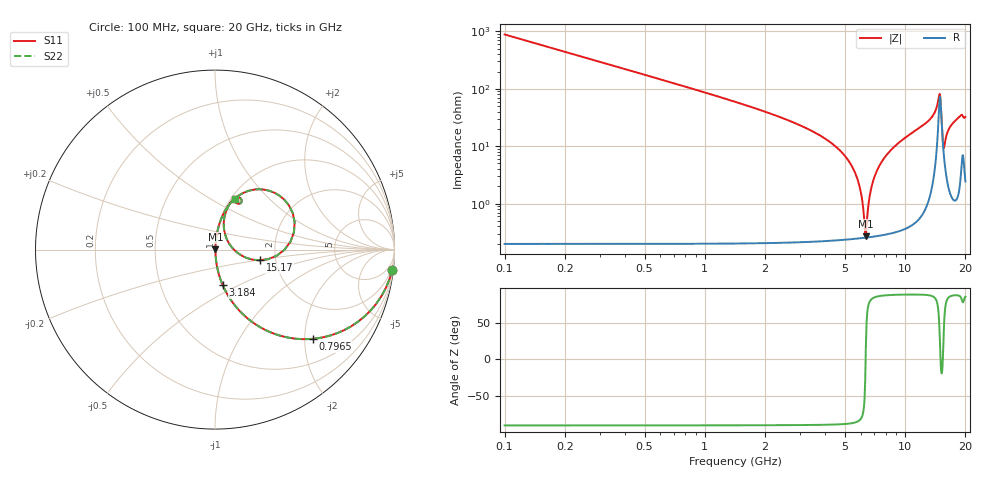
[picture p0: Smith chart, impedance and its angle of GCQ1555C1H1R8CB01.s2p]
!Murata Part Number: GCQ1555C1H1R8CB01
!These Parameters are Measured in Series Mode Connection
!Data Generated on Jan 08, 2026
!  o--ll--o
!Port1  Port2
!  o------o
!Operation Temp=25[degC], DC Bias Voltage=0[V]
!Freq. Start=100[MHz] Stop=20[GHz] 401[Steps]
# Hz S RI R 50
!Freq.(Hz) S11(Real) S11(Imag) S21(Real) S21(Imag) S12(Real) S12(Imag) S22(Real) S22(Imag)
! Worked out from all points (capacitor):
!   401 points, 100 MHz to 20 GHz, reference 50 ohm
!   read as one part in series: C = 1.8 pF near 199.5 MHz
!   lowest |Z| = 268 mohm at 6.369 GHz (marker M1)
!   series resonance near 6.351 GHz, so ESL is about 350 pH
!   S11 on the Smith chart (normalised r, x): 100 MHz: 1, -18; 796.5 MHz: 1.00, -2.19; 3.184 GHz: 1.00, -0.42; 15.17 GHz: 1.65, -0.21; 20 GHz: 1.05, +0.65
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1e8  0.9873 -0.1117  0.0127 0.1117  0.0127 0.1117  0.9873 -0.1117
3.985e8  0.8299 -0.3753  0.1701 0.3753  0.1701 0.3753  0.8299 -0.3753
7.965e8  0.5442 -0.4971  0.4558 0.4971  0.4558 0.4971  0.5442 -0.4971
1.692e9  0.1921 -0.3919  0.8079 0.3919  0.8079 0.3919  0.1921 -0.3919
3.1845e9  0.0436 -0.1992  0.9564 0.1992  0.9564 0.1992  0.0436 -0.1992
3.43325e9  0.0344 -0.1765  0.9656 0.1765  0.9656 0.1765  0.0344 -0.1765
4.72675e9  0.00931 -0.0833  0.9907 0.0833  0.9907 0.0833  0.00931 -0.0833
5.52275e9  0.00397 -0.0393  0.996 0.0393  0.996 0.0393  0.00397 -0.0393
5.9705e9  0.00279 -0.0174  0.9972 0.0174  0.9972 0.0174  0.00279 -0.0174
6.269e9  0.00254 -0.00365  0.9975 0.00365  0.9975 0.00365  0.00254 -0.00365
6.3685e9  0.00255 0.000794  0.9975 -0.000794  0.9975 -0.000794  0.00255 0.000794
6.7665e9  0.00294 0.018  0.9971 -0.018  0.9971 -0.018  0.00294 0.018
7.21425e9  0.00403 0.0363  0.996 -0.0363  0.996 -0.0363  0.00403 0.0363
7.861e9  0.00663 0.0613  0.9934 -0.0613  0.9934 -0.0613  0.00663 0.0613
1.005e10  0.0232 0.1381  0.9768 -0.1381  0.9768 -0.1381  0.0232 0.1381
1.338325e10  0.0939 0.2684  0.9061 -0.2684  0.9061 -0.2684  0.0939 0.2684
1.457725e10  0.306 0.3268  0.694 -0.3268  0.694 -0.3268  0.306 0.3268
1.487575e10  0.4437 0.1526  0.5563 -0.1526  0.5563 -0.1526  0.4437 0.1526
1.517425e10  0.2509 -0.0596  0.7491 0.0596  0.7491 0.0596  0.2509 -0.0596
1.557225e10  0.0735 0.0426  0.9265 -0.0426  0.9265 -0.0426  0.0735 0.0426
1.67165e10  0.0568 0.1976  0.9432 -0.1976  0.9432 -0.1976  0.0568 0.1976
2e10  0.1118 0.2798  0.8882 -0.2798  0.8882 -0.2798  0.1118 0.2798
